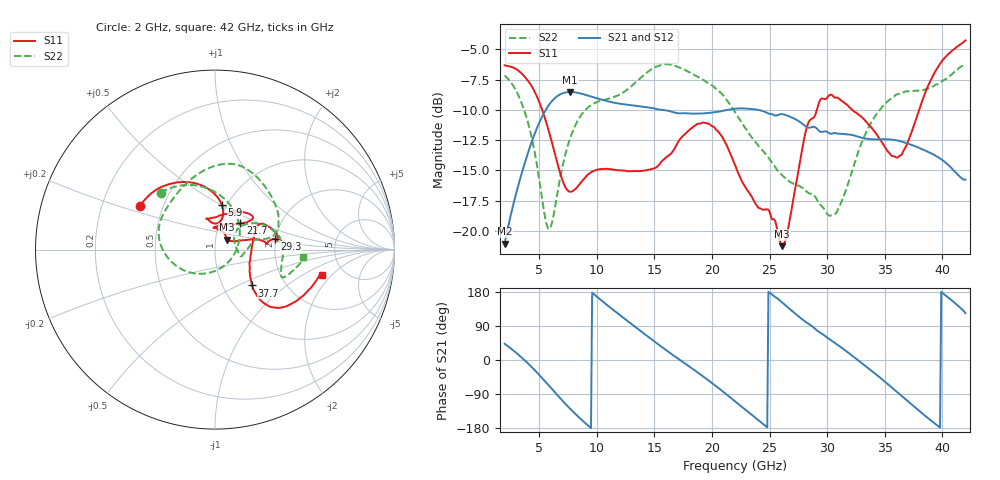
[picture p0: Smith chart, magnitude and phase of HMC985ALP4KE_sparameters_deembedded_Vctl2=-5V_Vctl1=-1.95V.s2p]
!s2p File: Measurements: S11, S21, S12, S22
# GHz S dB R 50.0
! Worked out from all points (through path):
!   401 points, 2 GHz to 42 GHz, reference 50 ohm
!   highest |S21| = -8.52 dB at 7.7 GHz (marker M1); lowest = -21.1 dB at 2 GHz (marker M2)
!   lowest |S11| = -21.3 dB at 26.1 GHz (marker M3), VSWR 1.19, Z = 56.8 + j6.23 ohm
!   |S11| at or under -10 dB: 5.259 GHz to 29.11 GHz (23.85 GHz wide, 139 % of centre); 32.19 GHz to 37.98 GHz (5.797 GHz wide, 16.5 % of centre)
!   |S22| runs from -19.9 to -6.2 dB; largest |S21 - S12| = 0.0004
!   S11 on the Smith chart (normalised r, x): 2 GHz: 0.37, +0.24; 5.9 GHz: 0.95, +0.50; 21.7 GHz: 1.26, +0.39; 29.3 GHz: 1.98, +0.27; 37.7 GHz: 1.37, -0.60; 42 GHz: 3.42, -1.53
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2  -6.32 149.6  -21.07 42.9  -21.07 42.9  -7.15 133.7
3.2  -6.76 130.6  -16.21 14.0  -16.21 14.0  -8.81 103.2
4.4  -8.13 108.3  -12.52 -20.1  -12.53 -20.1  -12.51 62.6
5.9  -11.97 81.3  -9.53 -69.6  -9.53 -69.6  -19.85 -50.5
7.7  -16.78 88.9  -8.52 -129.0  -8.53 -129.0  -12.31 -160.6
8.7  -15.92 100.3  -8.67 -158.2  -8.67 -158.2  -10.36 175.0
10.2  -14.91 104.3  -9.10 162.3  -9.10 162.3  -9.29 152.8
12.2  -15.02 105.5  -9.52 113.9  -9.52 113.9  -8.61 127.5
15.4  -14.55 84.5  -9.98 40.0  -9.98 40.0  -6.34 82.6
18.4  -11.39 49.2  -10.31 -25.0  -10.31 -24.9  -7.08 48.7
21.7  -13.84 46.0  -9.95 -101.7  -9.95 -101.6  -9.73 12.8
22  -14.55 50.3  -9.91 -109.1  -9.91 -109.1  -10.19 12.1
24.1  -18.14 90.9  -10.02 -160.6  -10.02 -160.6  -13.06 12.9
26.1  -21.27 39.1  -10.36 151.6  -10.36 151.6  -15.43 -3.6
28.7  -10.72 6.1  -11.41 89.0  -11.42 89.0  -16.95 -11.4
29.3  -9.38 10.0  -11.75 74.0  -11.75 74.0  -17.73 -6.3
30.7  -9.00 13.0  -11.91 44.4  -11.91 44.5  -18.61 24.1
32.4  -10.18 26.9  -12.14 6.1  -12.14 6.1  -14.38 42.0
35.4  -13.57 7.2  -12.45 -67.2  -12.44 -67.1  -9.19 17.0
37.7  -10.83 -44.0  -13.03 -126.9  -13.03 -126.9  -8.41 -6.6
39.8  -6.18 -41.2  -14.02 -178.3  -14.02 -178.2  -7.72 -22.1
42  -4.26 -13.3  -15.76 123.5  -15.76 123.6  -6.18 -5.0
